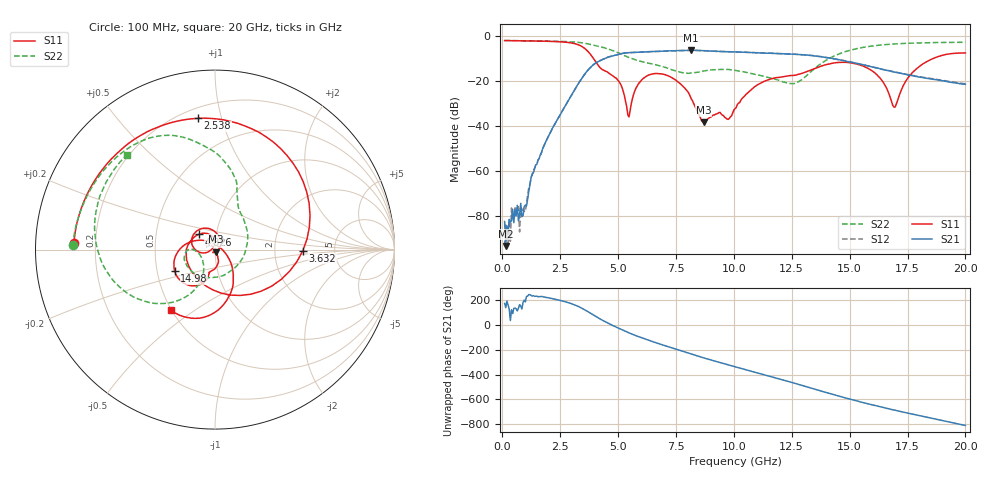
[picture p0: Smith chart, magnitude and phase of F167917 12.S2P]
!  2-Port S-parameters saved by WinCal
! VAR MeasName=S-Parameters (CALIBRATED_DATA) read from VNA (N5242A)
! VAR MeasDate=2016-11-22 9:00:15
! VAR NAME=F167917 12
! VAR FILENAME=F167917 12.S2P
! VAR DATE=2016-11-22 9:00:15
! VAR PHYS_PORTS=1,2
# Hz S DB R 50
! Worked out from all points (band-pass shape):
!   401 points, 100 MHz to 20 GHz, reference 50 ohm
!   highest |S21| = -6.40 dB at 8.159 GHz (marker M1); lowest = -93.2 dB at 149.8 MHz (marker M2)
!   |S21| within 3 dB of the highest: 4.575 GHz to 13.86 GHz (9.28 GHz wide, 101 % of centre)
!   lowest |S11| = -38.4 dB at 8.707 GHz (marker M3), VSWR 1.02, Z = 50.5 - j1.09 ohm
!   |S11| at or under -10 dB: 3.934 GHz to 18.62 GHz (14.68 GHz wide, 130 % of centre)
!   |S22| runs from -21.2 to -2.0 dB; largest |S21 - S12| = 0.0034
!   S11 on the Smith chart (normalised r, x): 100 MHz: 0.12, +0.02; 2.538 GHz: 0.26, +0.84; 3.632 GHz: 2.92, -0.04; 4.826 GHz: 0.82, +0.14; 14.98 GHz: 0.62, -0.16; 20 GHz: 0.50, -0.41
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1e8  -2.08 177.3  -82.41 175.9  -93.37 5.6  -2.03 178.3
1.4975e8  -2.09 176.0  -93.23 140.9  -83.51 169.9  -2.03 177.5
9.4575e8  -2.21 154.7  -75.77 -157.6  -77.88 -149.7  -2.16 164.7
1.34375e9  -2.28 143.3  -60.82 -121.8  -59.62 -123.7  -2.23 158.4
2.53775e9  -2.64 97.4  -34.33 -162.0  -34.31 -162.6  -2.47 137.0
3.43325e9  -4.68 26.0  -18.85 136.9  -18.87 136.9  -3.07 115.4
3.63225e9  -6.20 -0.6  -16.02 116.2  -16.02 116.3  -3.40 109.9
4.279e9  -14.64 -126.6  -10.74 43.7  -10.70 43.5  -4.95 93.7
4.82625e9  -18.16 137.1  -8.74 -8.3  -8.73 -8.6  -6.73 79.7
5.473e9  -36.00 160.1  -7.45 -62.9  -7.43 -63.1  -9.60 68.1
5.9705e9  -20.13 -174.8  -7.15 -99.2  -7.15 -99.4  -11.29 61.7
6.7665e9  -16.74 137.0  -6.83 -150.8  -6.84 -151.0  -13.21 38.9
8.1595e9  -27.92 39.4  -6.40 126.1  -6.41 126.0  -16.48 -68.8
8.70675e9  -38.43 -64.7  -6.57 94.2  -6.58 94.2  -15.57 -112.8
1.005e10  -32.29 -75.1  -7.13 22.8  -7.13 22.9  -15.31 -170.0
1.189075e10  -18.47 -99.1  -7.83 -72.2  -7.79 -72.1  -19.56 -174.7
1.338325e10  -14.92 -106.3  -8.75 -152.6  -8.72 -152.4  -15.39 -114.8
1.497525e10  -11.86 -151.7  -11.55 122.8  -11.48 122.7  -6.50 -141.6
1.67165e10  -26.21 121.2  -15.50 41.1  -15.53 41.8  -3.73 -178.6
1.696525e10  -31.60 42.2  -16.18 30.5  -16.04 31.2  -3.56 176.9
1.805975e10  -13.20 -62.6  -18.34 -14.4  -18.20 -13.7  -3.09 159.2
2e10  -7.57 -125.9  -21.49 -92.4  -21.28 -92.8  -2.85 133.0
